ORGANIZATION_BLOCK OB 1
BEGIN

	// Start timer and let it expire
	__STWRST
	L		0
	SS		T 10
	SET
	R		T 10
	U		T 10
	__ASSERT==	__STW VKE,	0
	SET
	L		W#16#0010
	SS		T 10
	U		T 10
	__ASSERT==	__STW VKE,	0
	L		T 10
	__ASSERT>=	__ACCU 1,	5
	__SLEEP		101
	U		T 10
	__ASSERT==	__STW VKE,	1
	L		T 10
	__ASSERT==	__ACCU 1,	0


	// Start timer and reset VKE before it expires
	__STWRST
	L		0
	SS		T 10
	SET
	R		T 10
	U		T 10
	__ASSERT==	__STW VKE,	0
	SET
	L		W#16#0010
	SS		T 10
	U		T 10
	__ASSERT==	__STW VKE,	0
	L		T 10
	__ASSERT>=	__ACCU 1,	5
	CLR
	L		W#16#0010
	SS		T 10
	U		T 10
	__ASSERT==	__STW VKE,	0
	L		T 10
	__ASSERT>=	__ACCU 1,	5
	__SLEEP		101
	U		T 10
	__ASSERT==	__STW VKE,	1
	L		T 10
	__ASSERT==	__ACCU 1,	0


	// Start timer and reset VKE after it expired
	__STWRST
	L		0
	SS		T 10
	SET
	R		T 10
	U		T 10
	__ASSERT==	__STW VKE,	0
	SET
	L		W#16#0010
	SS		T 10
	U		T 10
	__ASSERT==	__STW VKE,	0
	__SLEEP		101
	U		T 10
	__ASSERT==	__STW VKE,	1
	CLR
	SS		T 10
	U		T 10
	__ASSERT==	__STW VKE,	1
	__SLEEP		101
	U		T 10
	__ASSERT==	__STW VKE,	1
	SET
	SS		T 10
	U		T 10
	__ASSERT==	__STW VKE,	1


	// Reset signal
	__STWRST
	L		0
	SS		T 10
	SET
	R		T 10
	U		T 10
	__ASSERT==	__STW VKE,	0
	SET
	L		W#16#0010
	SS		T 10
	U		T 10
	__ASSERT==	__STW VKE,	0
	L		T 10
	__ASSERT>=	__ACCU 1,	5
	SET
	R		T 10
	U		T 10
	__ASSERT==	__STW VKE,	0
	L		T 10
	__ASSERT==	__ACCU 1,	0
	__SLEEP		101
	U		T 10
	__ASSERT==	__STW VKE,	0
	L		T 10
	__ASSERT==	__ACCU 1,	0


	// Test timer parameter
	AUF		DB 1
	L		DBW 0
	__ASSERT==	__ACCU 1,	24
	CALL FB 1, DB 1 (
		TIMER_VAR	:= T 42
	)


	CALL SFC 46 // STOP CPU
END_ORGANIZATION_BLOCK


FUNCTION_BLOCK FB 1
	VAR_INPUT
		TIMER_VAR	: TIMER
	END_VAR
BEGIN
	L		DIW 0
	__ASSERT==	__ACCU 1,	42
	L		#TIMER_VAR
	__ASSERT==	__ACCU 1,	0
	U		#TIMER_VAR
	__ASSERT==	__STW VKE,	0

	SS		#TIMER_VAR
END_FUNCTION_BLOCK


DATA_BLOCK DB 1
	FB 1
BEGIN
	TIMER_VAR	:= T 24
END_DATA_BLOCK
